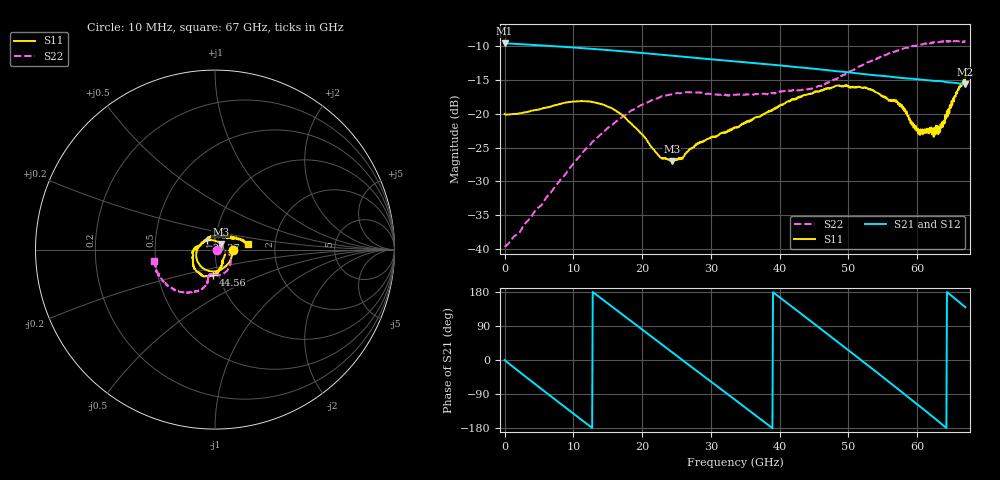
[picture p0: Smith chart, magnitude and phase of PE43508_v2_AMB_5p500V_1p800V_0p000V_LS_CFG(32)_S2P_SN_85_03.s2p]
!Keysight Technologies,N5227A,US51270237,A.10.43.00
!Date: Wednesday, August 22, 2018 17:09:53
!Correction: S11(Full 2 Port(1,3))
!S31(Full 2 Port(1,3))
!S13(Full 2 Port(1,3))
!S33(Full 2 Port(1,3))
!S2P File: Measurements: S11, S31, S13, S33:
# Hz S  dB  R 50
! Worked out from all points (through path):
!   801 points, 10 MHz to 67 GHz, reference 50 ohm
!   highest |S21| = -9.53 dB at 10 MHz (marker M1); lowest = -15.6 dB at 66.92 GHz (marker M2)
!   group delay of S21, straight-line fit = 38.7 ps
!   lowest |S11| = -27.0 dB at 24.29 GHz (marker M3), VSWR 1.09, Z = 53.1 + j3.35 ohm
!   |S11| at or under -10 dB: start of sweep to end of sweep
!   |S22| runs from -39.6 to -9.1 dB; largest |S21 - S12| = 0.0018
!   S11 on the Smith chart (normalised r, x): 10 MHz: 1.22, -0.00; 20.27 GHz: 0.91, +0.09; 44.56 GHz: 0.94, -0.27; 67 GHz: 1.45, +0.10
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1e7  -20.03 -0.6  -9.53 -0.2  -9.53 -0.2  -39.61 -1.3
2.522125e9  -19.87 -25.3  -9.69 -36.4  -9.69 -36.4  -37.05 15.5
5.70415e9  -19.16 -56.0  -9.88 -81.3  -9.88 -81.2  -33.02 21.8
8.300012e9  -18.48 -82.5  -10.06 -117.6  -10.05 -117.6  -29.57 18.3
1.123082e10  -18.12 -113.1  -10.26 -158.4  -10.27 -158.4  -25.91 4.9
1.499901e10  -18.94 -155.8  -10.56 149.3  -10.56 149.4  -22.12 -14.2
1.776235e10  -20.82 169.9  -10.79 111.2  -10.78 111.2  -20.05 -29.6
2.027448e10  -23.34 131.0  -11.01 76.5  -11.01 76.5  -18.53 -43.8
2.236791e10  -26.16 89.2  -11.21 47.7  -11.20 47.7  -17.63 -56.1
2.429388e10  -27.03 44.9  -11.39 21.3  -11.38 21.3  -17.14 -66.4
2.956934e10  -23.73 -35.9  -11.88 -51.0  -11.88 -51.0  -17.01 -88.8
3.3505e10  -22.08 -58.9  -12.23 -104.9  -12.23 -104.9  -17.19 -96.7
3.88642e10  -19.57 -73.4  -12.71 -178.8  -12.72 -178.8  -16.95 -101.4
4.455835e10  -17.07 -94.0  -13.28 102.0  -13.27 102.0  -16.29 -103.7
4.472582e10  -16.98 -95.4  -13.29 99.6  -13.28 99.6  -16.25 -103.8
5.067119e10  -16.09 -125.0  -13.95 16.2  -13.93 16.2  -13.53 -105.2
5.586291e10  -18.09 -164.7  -14.47 -57.5  -14.46 -57.8  -11.05 -121.2
5.787261e10  -19.26 175.6  -14.70 -86.3  -14.71 -86.5  -10.39 -128.9
6.021726e10  -22.37 141.6  -14.89 -120.0  -14.90 -120.3  -9.81 -138.3
6.272939e10  -21.78 83.7  -15.13 -156.6  -15.14 -156.9  -9.38 -149.8
6.691626e10  -15.13 13.0  -15.60 140.4  -15.68 140.4  -9.24 -168.9
6.7e10  -14.60 10.1  -15.60 139.0  -15.68 139.0  -9.30 -169.8
